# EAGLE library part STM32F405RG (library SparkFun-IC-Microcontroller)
STM32F405RGT6 ARM DSP Chip used on the WAV Trigger board. IC MCU 32BIT 1MB FLASH 64LQFP Datasheet SparkFun Products WAV Trigger (WIG-13660)
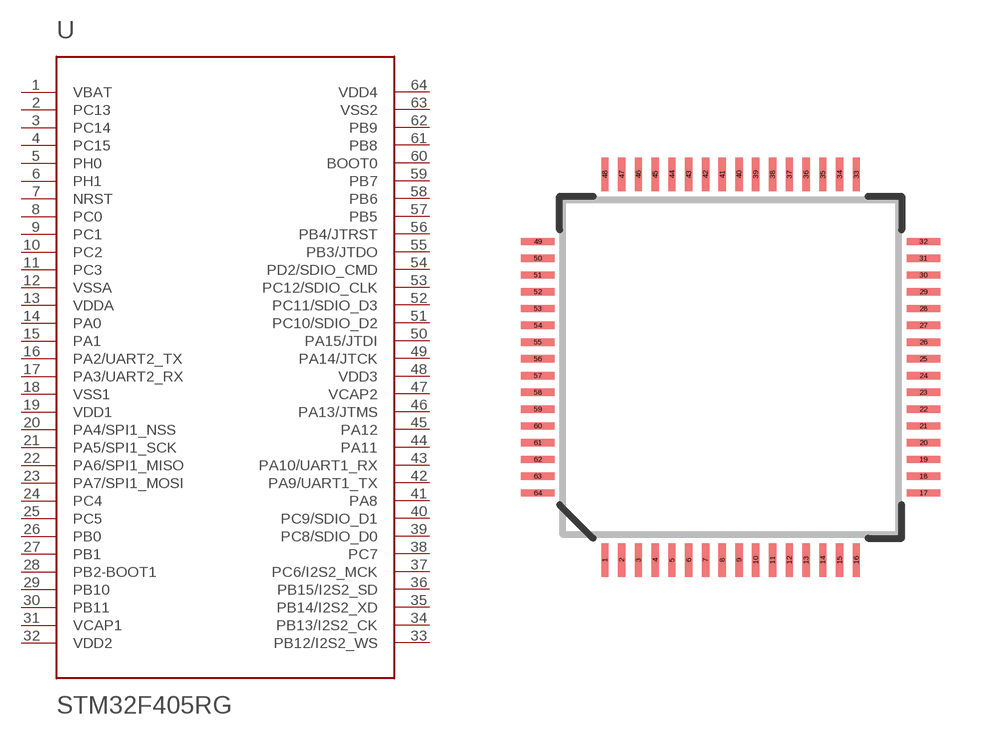
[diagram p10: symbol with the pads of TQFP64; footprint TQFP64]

Designator prefix -

## STM32F405RG (PROD_ID: IC-11709; VALUE: STM32F405RGT6)  [TQFP64]
1  VBAT
2  PC13
3  PC14
4  PC15
5  PH0
6  PH1
7  NRST
8  PC0
9  PC1
10  PC2
11  PC3
12  VSSA
13  VDDA
14  PA0
15  PA1
16  PA2/UART2_TX
17  PA3/UART2_RX
18  VSS1
19  VDD1
20  PA4/SPI1_NSS
21  PA5/SPI1_SCK
22  PA6/SPI1_MISO
23  PA7/SPI1_MOSI
24  PC4
25  PC5
26  PB0
27  PB1
28  PB2-BOOT1
29  PB10
30  PB11
31  VCAP1
32  VDD2
33  PB12/I2S2_WS
34  PB13/I2S2_CK
35  PB14/I2S2_XD
36  PB15/I2S2_SD
37  PC6/I2S2_MCK
38  PC7
39  PC8/SDIO_D0
40  PC9/SDIO_D1
41  PA8
42  PA9/UART1_TX
43  PA10/UART1_RX
44  PA11
45  PA12
46  PA13/JTMS
47  VCAP2
48  VDD3
49  PA14/JTCK
50  PA15/JTDI
51  PC10/SDIO_D2
52  PC11/SDIO_D3
53  PC12/SDIO_CLK
54  PD2/SDIO_CMD
55  PB3/JTDO
56  PB4/JTRST
57  PB5
58  PB6
59  PB7
60  BOOT0
61  PB8
62  PB9
63  VSS2
64  VDD4

## Footprint TQFP64 (pad centres in mm)
64-Lead TQFP Plastic Thin Quad Flatpack - 10x10x1mm Body, 2mmFP
smd 0.22 x 1: 1 -3.75,-5.75; 2 -3.25,-5.75; 3 -2.75,-5.75; 4 -2.25,-5.75; 5 -1.75,-5.75; 6 -1.25,-5.75; 7 -0.75,-5.75; 8 -0.25,-5.75; 9 0.25,-5.75; 10 0.75,-5.75; 11 1.25,-5.75; 12 1.75,-5.75; 13 2.25,-5.75; 14 2.75,-5.75; 15 3.25,-5.75; 16 3.75,-5.75; 33 3.75,5.75; 34 3.25,5.75; 35 2.75,5.75; 36 2.25,5.75; 37 1.75,5.75; 38 1.25,5.75; 39 0.75,5.75; 40 0.25,5.75; 41 -0.25,5.75; 42 -0.75,5.75; 43 -1.25,5.75; 44 -1.75,5.75; 45 -2.25,5.75; 46 -2.75,5.75; 47 -3.25,5.75; 48 -3.75,5.75
smd 1 x 0.22: 17 5.75,-3.75; 18 5.75,-3.25; 19 5.75,-2.75; 20 5.75,-2.25; 21 5.75,-1.75; 22 5.75,-1.25; 23 5.75,-0.75; 24 5.75,-0.25; 25 5.75,0.25; 26 5.75,0.75; 27 5.75,1.25; 28 5.75,1.75; 29 5.75,2.25; 30 5.75,2.75; 31 5.75,3.25; 32 5.75,3.75; 49 -5.75,3.75; 50 -5.75,3.25; 51 -5.75,2.75; 52 -5.75,2.25; 53 -5.75,1.75; 54 -5.75,1.25; 55 -5.75,0.75; 56 -5.75,0.25; 57 -5.75,-0.25; 58 -5.75,-0.75; 59 -5.75,-1.25; 60 -5.75,-1.75; 61 -5.75,-2.25; 62 -5.75,-2.75; 63 -5.75,-3.25; 64 -5.75,-3.75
